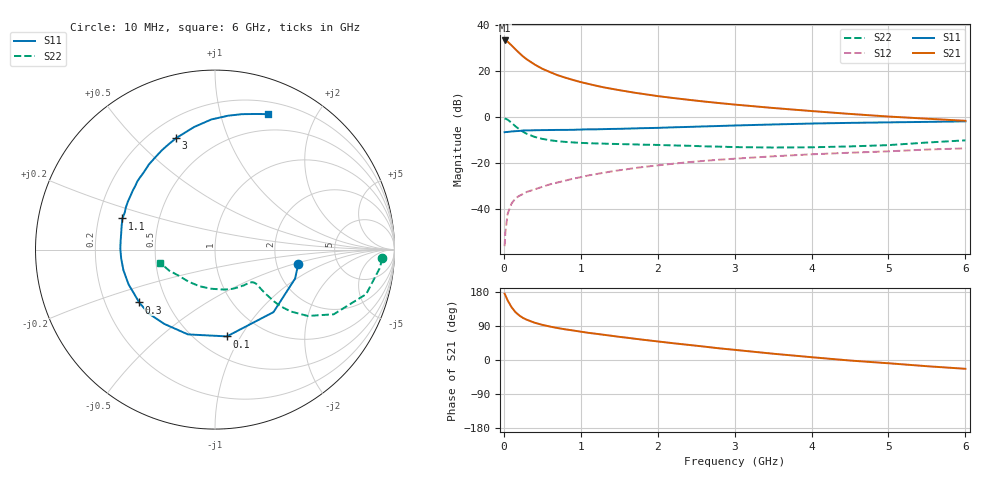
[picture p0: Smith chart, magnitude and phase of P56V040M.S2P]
! SIEMENS Small Signal Semiconductors
! BFP183
! Si NPN RF Bipolar Junction Transistor in SOT143
! VCE = 6 V  IC = 40 mA
! Common Emitter S-Parameters:  March  1996
# GHz  S  MA  R  50
!  f  S11  S21  S12  S22
! GHz  MAG  ANG  MAG  ANG  MAG  ANG  MAG  ANG
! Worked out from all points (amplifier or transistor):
!   36 points, 10 MHz to 6 GHz, reference 50 ohm
!   highest |S21| = 33.2 dB at 10 MHz (marker M1)
!   |S21| within 3 dB of that: start of sweep to 126.2 MHz
!   unconditionally stable (mu >= 1): 619.5 MHz to 5.8 GHz
!   at 250 MHz: K = 0.62, MSG = 29.8 dB, |S12| = -33.3 dB
!   at 1.4 GHz: K = 1.17, MAG = 15.4 dB, |S12| = -23.5 dB
!   at 6 GHz: K = 0.98, MSG = 6.0 dB, |S12| = -13.5 dB
!   S11 on the Smith chart (normalised r, x): 10 MHz: 2.66, -0.53; 100 MHz: 0.69, -0.87; 300 MHz: 0.35, -0.28; 1.1 GHz: 0.30, +0.15; 3 GHz: 0.30, +0.67; 6 GHz: 0.32, +1.41
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0.01  0.471 -9.5  45.76 174.9  0.0016 87.2  0.9334 -3.0
0.02  0.4745 -19.9  45.49 170.6  0.0032 85.0  0.9231 -6.5
0.05  0.477 -46.9  42.96 157.1  0.0081 76.8  0.8782 -16.4
0.1  0.4881 -82.2  35.87 139.4  0.0134 60.9  0.7531 -28.6
0.15  0.4959 -107.7  29.53 126.5  0.0173 55.0  0.6349 -35.6
0.2  0.5013 -124.3  24.51 117.6  0.0197 53.0  0.5455 -39.2
0.25  0.5135 -136.3  20.6 110.9  0.0217 52.0  0.4811 -40.9
0.3  0.5147 -145.1  17.78 106.1  0.024 51.2  0.4332 -41.3
0.4  0.5191 -158.1  13.81 98.4  0.0272 52.8  0.3731 -41.1
0.5  0.523 -167.3  11.16 92.8  0.0309 53.6  0.3375 -40.6
0.6  0.525 -174.4  9.444 88.2  0.035 55.6  0.3151 -40.0
0.7  0.5276 179.5  8.083 84.3  0.0384 56.7  0.3004 -39.8
0.8  0.5281 174.5  7.144 80.9  0.0421 57.4  0.2907 -39.9
1  0.5372 165.4  5.732 74.7  0.05 57.9  0.2765 -41.2
1.1  0.5443 161.4  5.237 71.7  0.0545 57.7  0.2722 -42.0
1.5  0.557 148.2  3.839 61.1  0.0706 56.4  0.2605 -47.2
2.2  0.6006 127.8  2.594 44.3  0.0977 51.1  0.2435 -61.1
3  0.6579 109.2  1.869 26.8  0.1257 43.4  0.2241 -81.8
3.5  0.6928 99.7  1.577 16.6  0.1415 38.8  0.2193 -97.0
4.5  0.75 84.3  1.172 -1.4  0.1692 29.4  0.2319 -129.9
5.5  0.788 73.5  0.924 -16.4  0.1983 21.2  0.2812 -155.5
6  0.8097 68.8  0.832 -23.2  0.2104 16.6  0.314 -166.4
